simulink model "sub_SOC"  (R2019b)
settings: Solver=VariableStepAuto  StartTime=0.0  StopTime=10.0  RelTol=1e-3

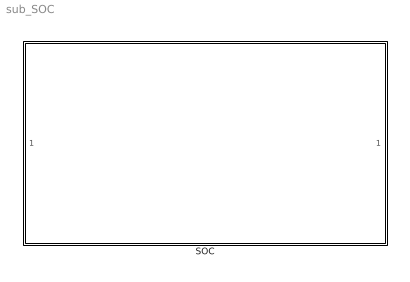
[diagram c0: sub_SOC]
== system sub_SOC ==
  SOC : Subsystem

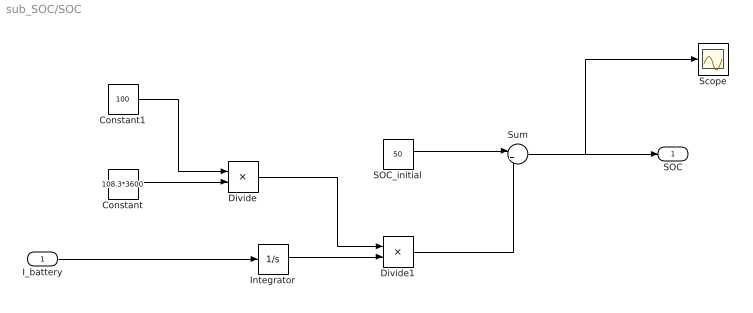
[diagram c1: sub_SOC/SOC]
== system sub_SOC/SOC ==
  I_battery : Inport
  Constant : Constant  Value=108.3*3600
  Constant1 : Constant  Value=100
  Divide : Product  Inputs=*/
  Divide1 : Product  Inputs=**
  Integrator : Integrator
  SOC_initial : Constant  Value=50
  Scope : Scope
  Sum : Sum  Inputs=|+-
  SOC : Outport
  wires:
  Constant/1 -> Divide/2
  Constant1/1 -> Divide/1
  I_battery/1 -> Integrator/1
  Divide/1 -> Divide1/1
  Integrator/1 -> Divide1/2
  SOC_initial/1 -> Sum/1
  Divide1/1 -> Sum/2
  Sum/1 -> Scope/1, SOC/1
